PROGRAM MAIN
VAR
	//ID:T_ULARGE_INTEGER ;
	Value:LREAL;

	fbDBCyclicRdWrt	: FB_DBCyclicRdWrt;
	bCyclic			: BOOL := TRUE;
	bBusy_Cyclic	: BOOL;
	bErr			: BOOL;
	nErrID			: UDINT;
	sSQLState		: ST_DBSQLError;
	
	ton1:ton;

END_VAR

ton1(IN:=NOT fbDBCyclicRdWrt.bBusy,pt:=T#10S );
IF ton1.Q THEN
	bCyclic:=TRUE;
END_IF

fbDBCyclicRdWrt(
	sNetID		:= ,
	bExecute	:= bCyclic,
	tTimeout	:= T#10S,
	bBusy		=> bBusy_Cyclic,
	bError		=> bErr,
	nErrID		=> nErrID,
	sSQLState	=> sSQLState);
IF NOT  fbDBCyclicRdWrt.bBusy THEN
	bCyclic:=FALSE;
END_IF

END_PROGRAM
